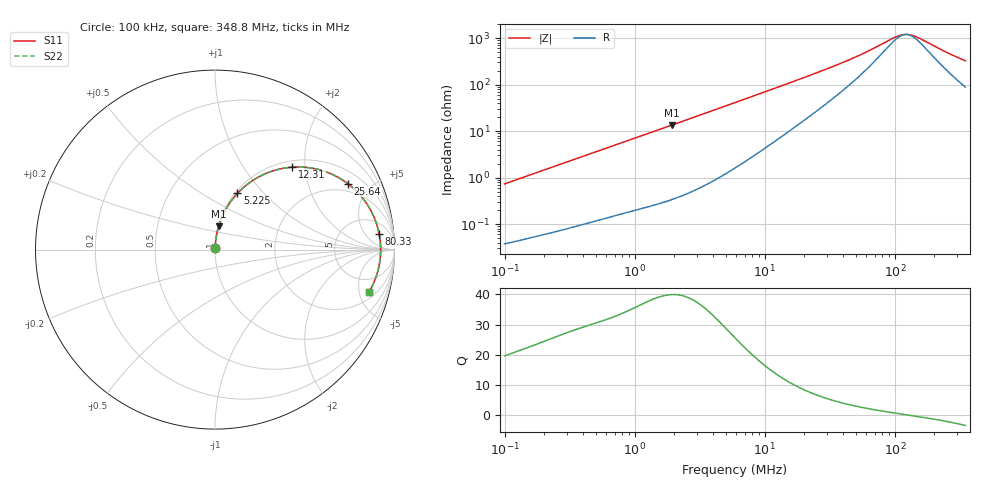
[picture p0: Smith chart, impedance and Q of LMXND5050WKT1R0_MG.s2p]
! LMXND5050WKT1R0_MG  S-PARAMETER MODEL  ( General Type )
! Model Generated by TAIYO YUDEN Corporation (https://www.yuden.co.jp/en/)
! Version 1.0
! TAIYO YUDEN Control No. 191023NI43SB-FBB
! Copyright(c) 2019 TAIYO YUDEN CO.,LTD. All Rights Reserved.
! Product Description (link to TY-COMPAS)
! https://ds.yuden.co.jp/TYCOMPAS/or/detail?pn=LMXND5050WKT1R0NMG&u=M
! Products Name : Inductors
! Characteristics :
!  Inductance : 1.0 uH , SRF(min) : 81 MHz , DC Resistance(max) : 0.0252 Ohm
!  Rated Current : Saturation :4000 mA , Temp Rise : 3600 mA (40 degC)
!  Case Size : 4.9 x 4.9 / 0.193 x 0.193 [mm/inch] , Thickness : 2 / 0.079 [mm/inch]
!  (Conditions: Temperature = 25 degC , DC Bias Current/Voltage = 0A / 0V)
! External Node Assignments :
!  1  o---GGG---o  2
! GND o---------o GND
! Frequency Range : 0.1MHz  -  348.750116MHz  [ 402 STEP ]
# MHz S RI R 50
! Freq[MHz].  S11 Real  S11 Imag  S21 Real  S21 Imag  S12 Real  S12 Imag  S22 Real  S22 Imag
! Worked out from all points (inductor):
!   401 points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, 100 kHz to 348.8 MHz, reference 50 ohm
!   read as one part in series: L = 1.16 uH near 104.2 kHz
!   highest Q = 39.9 at 1.924 MHz (marker M1), where L = 1.11 uH
!   self-resonance near 122.1 MHz
!   S11 on the Smith chart (normalised r, x): 100 kHz: 1.00, +0.01; 5.225 MHz: 1.03, +0.73; 12.31 MHz: 1.13, +1.71; 25.64 MHz: 1.57, +3.63; 80.33 MHz: 11, +12; 348.8 MHz: 2.76, -6.26
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0.1  0.000427 0.00731  0.9996 -0.00731  0.9996 -0.00731  0.000427 0.00731
0.392077  0.00174 0.0278  0.9983 -0.0278  0.9983 -0.0278  0.00174 0.0278
0.833784  0.00512 0.0582  0.9949 -0.0582  0.9949 -0.0582  0.00512 0.0582
1.537242  0.014 0.1053  0.986 -0.1053  0.986 -0.1053  0.014 0.1053
1.923807  0.0208 0.1306  0.9792 -0.1306  0.9792 -0.1306  0.0208 0.1306
3.40516  0.0585 0.2211  0.9415 -0.2211  0.9415 -0.2211  0.0585 0.2211
5.225399  0.125 0.3133  0.875 -0.3133  0.875 -0.3133  0.125 0.3133
5.905507  0.1536 0.3415  0.8464 -0.3415  0.8464 -0.3415  0.1536 0.3415
8.352453  0.2631 0.4151  0.7369 -0.4151  0.7369 -0.4151  0.2631 0.4151
12.30505  0.43 0.4594  0.57 -0.4594  0.57 -0.4594  0.43 0.4594
16.70813  0.5726 0.4472  0.4274 -0.4472  0.4274 -0.4472  0.5726 0.4472
23.15412  0.7058 0.391  0.2942 -0.391  0.2942 -0.391  0.7058 0.391
25.63951  0.7403 0.3673  0.2597 -0.3673  0.2597 -0.3673  0.7403 0.3673
34.11126  0.817 0.2939  0.183 -0.2939  0.183 -0.2939  0.817 0.2939
47.27139  0.8729 0.209  0.1271 -0.209  0.1271 -0.209  0.8729 0.209
80.32704  0.9149 0.086  0.0851 -0.086  0.0851 -0.086  0.9149 0.086
90.78195  0.9191 0.0603  0.0809 -0.0603  0.0809 -0.0603  0.9191 0.0603
113.6105  0.9228 0.0145  0.0772 -0.0145  0.0772 -0.0145  0.9228 0.0145
133.7423  0.9227 -0.0184  0.0773 0.0184  0.0773 0.0184  0.9227 -0.0184
154.2634  0.9206 -0.0474  0.0794 0.0474  0.0794 0.0474  0.9206 -0.0474
262.1358  0.8931 -0.1637  0.1069 0.1637  0.1069 0.1637  0.8931 -0.1637
348.7501  0.8589 -0.2347  0.1411 0.2347  0.1411 0.2347  0.8589 -0.2347
